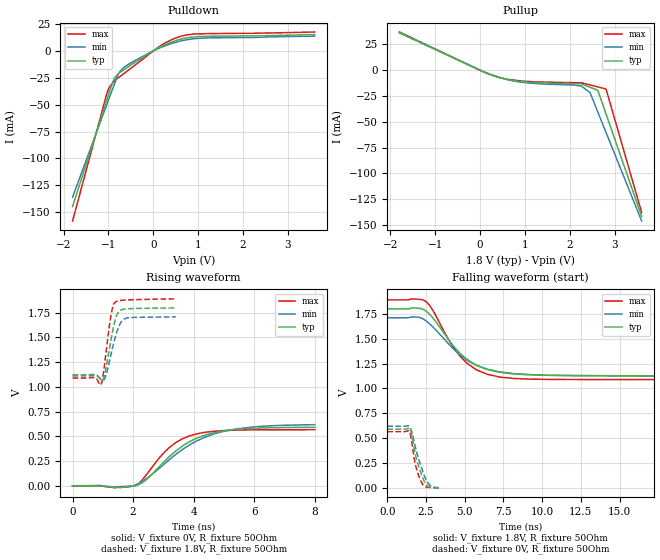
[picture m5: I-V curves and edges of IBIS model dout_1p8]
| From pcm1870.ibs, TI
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|   dout_1p8 Model
[Model]   dout_1p8
Model_type   Output
Polarity   Non-Inverting
Vmeas = 0.9
Vref = 0.9
Cref = 10pF
Rref = 50
|   typ   min   max
C_comp   8.600e-13   7.020e-13   9.095e-13
[Voltage Range]   1.8   1.71   1.89
|Ambient Temperature   25   85   -40
|Junction Temperature
[Temperature Range]   26   86   -40
[Pullup Reference]   1.8   1.71   1.89
[Pulldown Reference]   0   0   0
[Power Clamp Reference]   1.8   1.71   1.89
[GND Clamp Reference]   0   0   0
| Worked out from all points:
|   slope of the pulldown table from 0 to 0.27 V, typ, clamps not added: 45.5 ohm
|   slope of the pullup table from 0 to 0.27 V, typ, clamps not added: 57.1 ohm
|   falling waveform, V_fixture 1.8V, R_fixture 50Ohm: 20-80 % time 2.32ns typ, 2.61ns min, 2.04ns max; typ from 1.8 V to 1.12 V
|   rising waveform, V_fixture 0V, R_fixture 50Ohm: 20-80 % time 1.42ns typ, 1.75ns min, 1.06ns max; typ from 0 V to 0.591 V
|   rising waveform, V_fixture 1.8V, R_fixture 50Ohm: 20-80 % time 252ps typ, 305ps min, 207ps max; typ from 1.12 V to 1.8 V
|   falling waveform, V_fixture 0V, R_fixture 50Ohm: 20-80 % time 599ps typ, 694ps min, 464ps max; typ from 0.592 V to 0.003 V
[Pulldown]
|   Voltage   I(typ)   I(min)   I(max)
-1.8V     -144.7mA   -136mA     -158.2mA
-1.042V   -46.4mA    -50.43mA   -40.53mA
-1.008V   -41.99mA   -46.6mA    -36.19mA
-951.4mV  -34.76mA   -40.29mA   -32mA
-896.4mV  -27.94mA   -34.18mA   -29.31mA
-860.7mV  -25.26mA   -30.21mA   -27.56mA
-744.9mV  -19.98mA   -19.06mA   -23.84mA
-594.5mV  -15.74mA   -13.54mA   -19.08mA
178.8mV   4.002mA    3.456mA    5.307mA
636.2mV   11.21mA    9.555mA    13.93mA
1.117V    13.53mA    12.01mA    16.05mA
3.6V      15.21mA    13.83mA    17.62mA
[Pullup]
|   Voltage   I(typ)   I(min)   I(max)
-1.8V     36.35mA    36.24mA    37.04mA
21.6mV    -459.6uA   -437uA     -466.6uA
409.4mV   -6.636mA   -6.731mA   -6.841mA
718.2mV   -9.798mA   -10.2mA    -9.362mA
1.1V      -11.54mA   -12.47mA   -10.93mA
2.254V    -13.1mA    -15.25mA   -12.11mA
2.449V    -16.45mA   -21.69mA   -14.25mA
2.623V    -19.44mA   -40.42mA   -16.15mA
2.806V    -42.34mA   -60.24mA   -18.16mA
3.6V      -141.5mA   -146.1mA   -137.8mA
[Ramp]
R_load = 50
|   typ   min   max
dV/dt_r   0.355121/1.42836e-09   0.372608/1.77345e-09   0.339935/1.06e-09
dV/dt_f   0.406174/2.31644e-09   0.356347/2.61222e-09   0.480808/2.0435e-09
[Falling Waveform]
V_fixture = 1.8V
V_fixture_min = 1.71V
V_fixture_max = 1.89V
R_fixture = 50Ohm
|   Time   V(typ)   V(min)   V(max)
0s        1.8V       1.71V      1.89V
1.78ns    1.809V     1.718V     1.899V
2.443ns   1.783V     1.685V     1.878V
2.875ns   1.721V     1.628V     1.801V
4.286ns   1.424V     1.395V     1.409V
5.161ns   1.292V     1.283V     1.251V
6.472ns   1.192V     1.193V     1.141V
8.19ns    1.146V     1.149V     1.101V
20.97ns   1.126V     1.123V     1.09V
65ns      1.123V     1.116V     1.089V
[Rising Waveform]
V_fixture = 0V
V_fixture_min = 0V
V_fixture_max = 0V
R_fixture = 50Ohm
|   Time   V(typ)   V(min)   V(max)
0s        333pV      28.48nV    288.8pV
1.391ns   -14.3mV    -11.09mV   -21.16mV
2.042ns   -1.618mV   3.889mV    -1.991mV
2.381ns   48.04mV    60.01mV    88.22mV
3.214ns   299.2mV    267.7mV    391.4mV
3.614ns   397.1mV    362.3mV    472.3mV
4.014ns   467.8mV    438mV      517.6mV
4.698ns   537.7mV    525.2mV    550.7mV
5.498ns   572mV      577.6mV    562.3mV
8ns       590.6mV    617.2mV    566.3mV
[Rising Waveform]
V_fixture = 1.8V
V_fixture_min = 1.71V
V_fixture_max = 1.89V
R_fixture = 50Ohm
|   Time   V(typ)   V(min)   V(max)
0s        1.121V     1.11V      1.088V
729.9ps   1.124V     1.113V     1.093V
942.9ps   1.07V      1.075V     1.026V
1.049ns   1.106V     1.076V     1.207V
1.264ns   1.467V     1.319V     1.712V
1.337ns   1.582V     1.414V     1.815V
1.415ns   1.682V     1.505V     1.856V
1.59ns    1.775V     1.648V     1.873V
1.78ns    1.787V     1.695V     1.877V
3.414ns   1.797V     1.706V     1.888V
[Falling Waveform]
V_fixture = 0V
V_fixture_min = 0V
V_fixture_max = 0V
R_fixture = 50Ohm
|   Time   V(typ)   V(min)   V(max)
0s        591.9mV    621mV      566.6mV
1.427ns   595.3mV    620.4mV    568mV
1.57ns    534.9mV    569.8mV    467.5mV
1.707ns   424mV      483.2mV    328.4mV
1.832ns   325.6mV    398.5mV    224.8mV
1.981ns   240.3mV    316.6mV    144.7mV
2.188ns   145.6mV    214.2mV    63.54mV
2.482ns   43.21mV    92.2mV     12.68mV
2.762ns   10.19mV    26.04mV    5.945mV
3.335ns   3.119mV    4.173mV    2.477mV
